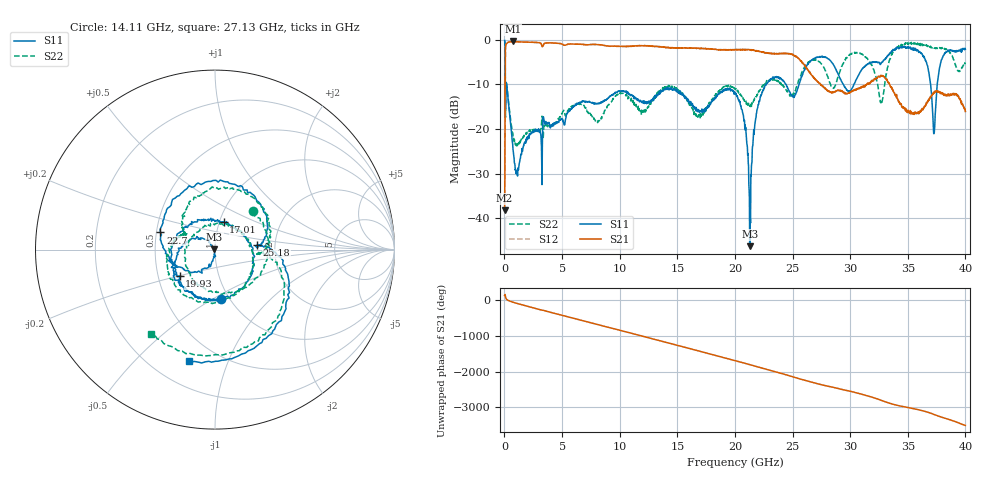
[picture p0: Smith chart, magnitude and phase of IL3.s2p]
!Agilent Technologies,N5230A,US43500312,A.07.50.67
!Agilent N5230A: A.07.50.67
!Date: Wednesday, December 30, 2015 20:09:47
!Correction: S11(Full 2 Port(1,2))
!S21(Full 2 Port(1,2))
!S12(Full 2 Port(1,2))
!S22(Full 2 Port(1,2))
!S2P File: Measurements: S11, S21, S12, S22:
# Hz S  dB  R 50
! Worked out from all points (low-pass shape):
!   1601 points, 10 MHz to 40 GHz, reference 50 ohm
!   highest |S21| = -0.31 dB at 709.8 MHz (marker M1); lowest = -38.2 dB at 10 MHz (marker M2)
!   |S21| within 3 dB of the highest: 79.56 MHz to 25.04 GHz (24.96 GHz wide, 199 % of centre)
!   lowest |S11| = -46.3 dB at 21.28 GHz (marker M3), VSWR 1.01, Z = 49.5 + j0.144 ohm
!   |S11| at or under -10 dB: 183.4 MHz to 22.7 GHz (22.52 GHz wide, 197 % of centre); 24.45 GHz to 25.56 GHz (1.112 GHz wide, 4.45 % of centre); 29.41 GHz to 30.32 GHz (906.8 MHz wide, 3.04 % of centre)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
!   |S22| runs from -24.0 to -0.2 dB; largest |S21 - S12| = 0.018
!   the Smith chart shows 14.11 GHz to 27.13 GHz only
!   S11 on the Smith chart (normalised r, x): 14.11 GHz: 0.91, -0.54; 17.01 GHz: 1.05, +0.33; 19.93 GHz: 0.65, -0.20; 22.7 GHz: 0.53, +0.11; 25.18 GHz: 1.60, +0.08; 27.13 GHz: 0.35, -0.73
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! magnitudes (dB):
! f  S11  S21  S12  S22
! 10 MHz  -0.1  -38.2  -38.5  -0.2
! 259.9 MHz  -11.9  -0.6  -0.6  -11.7
! 709.8 MHz  -23.4  -0.3  -0.3  -20.8
! 6.683 GHz  -13.9  -1.0  -1.0  -14.5
! 13.36 GHz  -12.0  -1.5  -1.6  -11.5
! 14.11 GHz  -11.1  -1.7  -1.6  -10.4
! 17.01 GHz  -15.9  -1.9  -1.9  -16.7
! 19.93 GHz  -12.2  -2.2  -2.2  -10.8
! 20 GHz  -11.9  -2.2  -2.2  -10.9
! 21.28 GHz  -46.3  -2.2  -2.2  -14.7
! 22.7 GHz  -9.9  -2.9  -2.8  -9.6
! 25.18 GHz  -12.6  -3.5  -3.6  -11.6
! 26.68 GHz  -4.5  -8.0  -8.1  -4.7
! 27.13 GHz  -3.9  -9.2  -9.3  -4.6
! 28.53 GHz  -5.5  -11.8  -11.7  -10.8
! 31.05 GHz  -6.6  -10.4  -10.4  -3.2
! 32.7 GHz  -5.2  -8.2  -8.1  -14.3
! 33.35 GHz  -3.3  -9.7  -9.6  -5.1
! 36.25 GHz  -3.1  -15.4  -15.4  -1.0
! 37.28 GHz  -21.0  -11.9  -11.7  -1.8
! 38.1 GHz  -3.5  -12.3  -12.2  -2.0
! 40 GHz  -2.1  -16.0  -16.1  -5.3
